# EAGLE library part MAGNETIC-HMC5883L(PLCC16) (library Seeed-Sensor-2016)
314040002
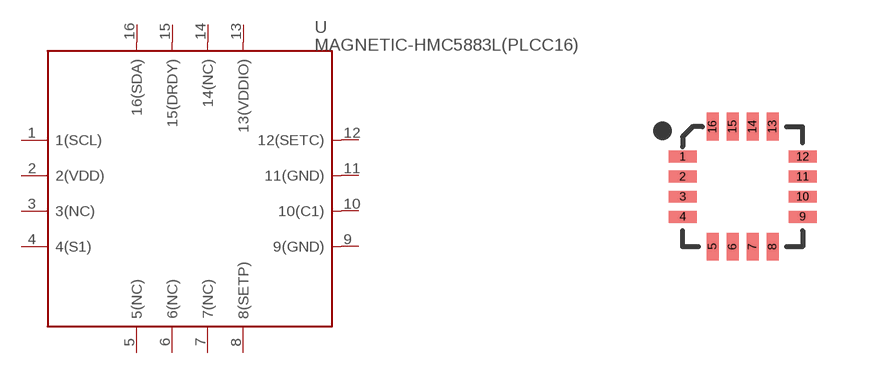
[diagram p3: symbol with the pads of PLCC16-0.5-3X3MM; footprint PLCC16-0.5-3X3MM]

Designator prefix U

## MAGNETIC-HMC5883L(PLCC16) (MPN: HMC5883L; VALUE: HMC5883L)  [PLCC16-0.5-3X3MM]
1  1(SCL)
2  2(VDD)  sup
3  3(NC)  nc
4  4(S1)
5  5(NC)  nc
6  6(NC)  nc
7  7(NC)  nc
8  8(SETP)
9  9(GND)  pwr
10  10(C1)
11  11(GND)  sup
12  12(SETC)
13  13(VDDIO)  sup
14  14(NC)  nc
15  15(DRDY)
16  16(SDA)

## Footprint PLCC16-0.5-3X3MM (pad centres in mm)
smd 0.7 x 0.3: 1 0,2.25; 2 0,1.75; 3 0,1.25; 4 0,0.75; 9 3,0.75; 10 3,1.25; 11 3,1.75; 12 3,2.25
smd 0.3 x 0.7: 5 0.75,0; 6 1.25,0; 7 1.75,0; 8 2.25,0; 13 2.25,3; 14 1.75,3; 15 1.25,3; 16 0.75,3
